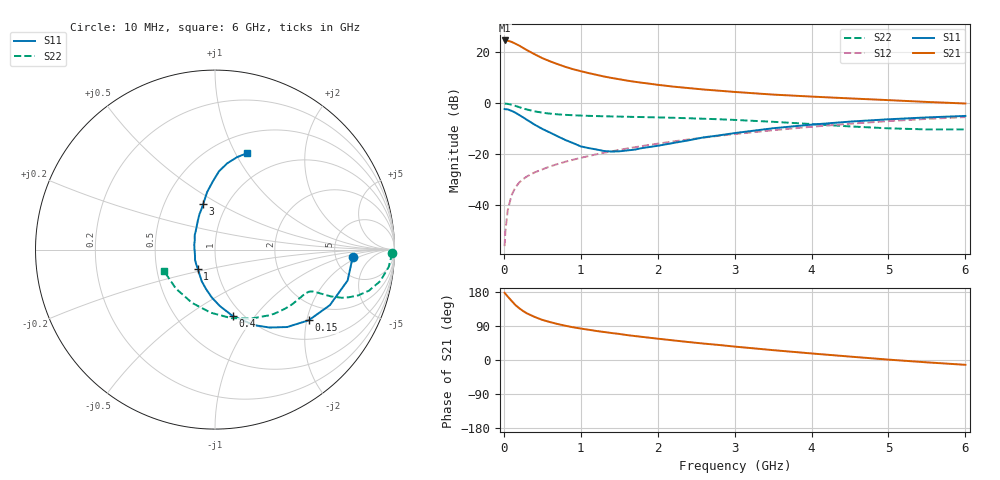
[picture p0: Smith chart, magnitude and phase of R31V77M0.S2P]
! SIEMENS Small Signal Semiconductors
! BFR181
! Si NPN RF Bipolar Junction Transistor in SOT23
! VCE = 1.75 V  IC = 7 mA
! Common Emitter S-Parameters:  May  1996
# GHz  S  MA  R  50
!  f  S11  S21  S12  S22
! GHz  MAG  ANG  MAG  ANG  MAG  ANG  MAG  ANG
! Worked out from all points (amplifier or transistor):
!   36 points, 10 MHz to 6 GHz, reference 50 ohm
!   highest |S21| = 24.6 dB at 10 MHz (marker M1)
!   |S21| within 3 dB of that: start of sweep to 254.9 MHz
!   unconditionally stable (mu >= 1): 840.2 MHz to 2.812 GHz
!   at 250 MHz: K = 0.53, MSG = 25.7 dB, |S12| = -29.7 dB
!   at 1.4 GHz: K = 1.08, MAG = 12.7 dB, |S12| = -18.8 dB
!   at 6 GHz: K = 0.86, MSG = 2.7 dB, |S12| = -5.4 dB
!   S11 on the Smith chart (normalised r, x): 10 MHz: 7.44, -1.43; 150 MHz: 1.49, -2.06; 400 MHz: 0.90, -0.78; 1 GHz: 0.81, -0.18; 3 GHz: 0.78, +0.42; 6 GHz: 0.70, +1.11
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0.01  0.7707 -2.9  16.93 177.4  0.0016 87.7  0.9861 -1.1
0.02  0.7644 -5.2  16.78 174.8  0.0031 88.4  0.9834 -2.3
0.05  0.7588 -13.1  16.79 167.6  0.008 84.1  0.9724 -5.7
0.1  0.711 -25.8  15.88 156.2  0.0158 77.0  0.9374 -10.8
0.15  0.6542 -37.0  14.64 145.2  0.0226 72.9  0.8882 -14.9
0.2  0.5898 -47.0  13.43 136.6  0.0281 69.6  0.8385 -17.7
0.25  0.5301 -55.0  12.1 129.3  0.0328 67.0  0.792 -19.6
0.3  0.4739 -62.6  10.94 123.1  0.037 66.0  0.7554 -20.8
0.4  0.382 -75.2  9.106 113.7  0.0443 64.6  0.6955 -22.0
0.5  0.315 -85.2  7.637 105.8  0.0508 65.0  0.6541 -22.4
0.6  0.2669 -93.9  6.616 100.1  0.0581 64.9  0.6266 -22.7
0.8  0.1911 -112.8  5.152 90.4  0.0717 65.8  0.5933 -23.2
1  0.1433 -132.1  4.239 83.0  0.0854 66.8  0.574 -24.1
1.1  0.1329 -142.1  3.898 79.9  0.0926 67.2  0.5673 -24.9
1.3  0.1165 -163.2  3.344 74.0  0.1075 67.0  0.5565 -26.5
1.6  0.1193 165.7  2.777 65.8  0.1303 66.5  0.5447 -29.6
2.2  0.1665 127.6  2.118 51.8  0.179 64.2  0.5197 -37.5
3  0.261 104.7  1.665 35.4  0.2495 58.6  0.4722 -51.0
3.5  0.3244 97.7  1.478 26.0  0.2969 54.1  0.4338 -62.5
4.5  0.4377 87.0  1.244 9.0  0.3979 43.2  0.3524 -93.8
5.5  0.5285 76.7  1.061 -6.2  0.494 30.0  0.3077 -135.2
6  0.5648 71.8  0.989 -12.7  0.5369 22.8  0.3083 -157.4
